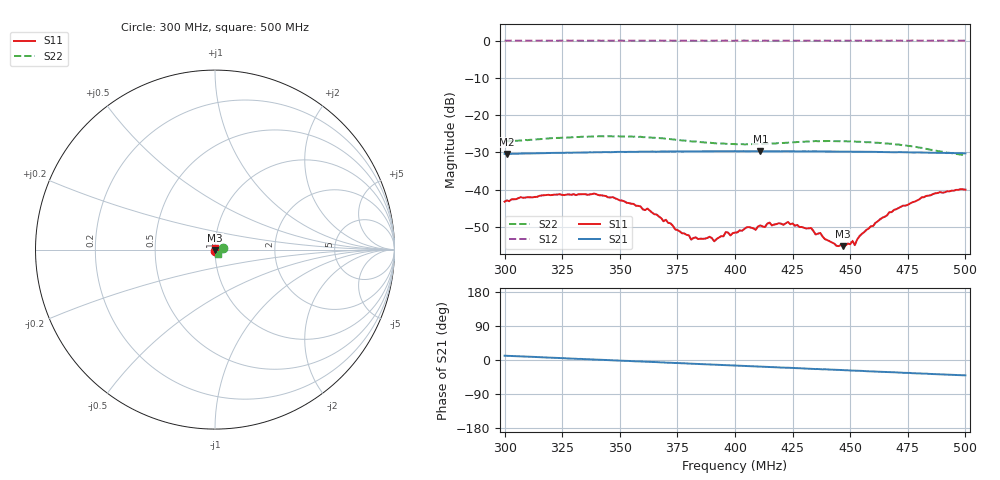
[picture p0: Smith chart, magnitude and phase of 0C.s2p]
!Prosund Technologies,SP809B,SP82221046,V.03.04.C
!Date: Monday, March 31, 2025 16:30:52
!Correction: S11(C* 2-Port  )
!S21(C* 2-Port  )
!S12(C* 2-Port  )
!S22(C* 2-Port  )
!S2P File: Measurement: :
# Hz S  dB  R 50
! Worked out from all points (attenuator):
!   201 points, 300 MHz to 500 MHz, reference 50 ohm
!   highest |S21| = -29.66 dB at 411 MHz (marker M1); lowest = -30.4 dB at 301 MHz (marker M2)
!   lowest |S11| = -55.2 dB at 447 MHz (marker M3), VSWR 1.00, Z = 50.1 - j0.142 ohm
!   |S11| at or under -10 dB: start of sweep to end of sweep
!   |S22| runs from -30.7 to -25.6 dB; largest |S21 - S12| = 0.98
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3e8  -43.21 -67.1  -30.41 11.3  0.01 0.0  -27.03 11.2
3.01e8  -42.88 -68.4  -30.41 11.1  -0.01 0.3  -27.01 10.9
3.34e8  -41.22 -52.1  -30.02 2.4  -0.02 0.1  -25.77 -0.6
3.47e8  -41.99 -32.2  -29.91 -0.9  -0.03 -0.0  -25.69 -1.5
3.62e8  -45.06 -2.5  -29.80 -4.7  -0.02 -0.2  -25.95 -2.8
3.67e8  -47.22 5.8  -29.78 -6.1  0.03 0.1  -26.15 -3.4
3.81e8  -53.41 58.6  -29.72 -9.7  -0.01 -0.3  -27.02 -8.0
3.89e8  -52.64 96.4  -29.70 -11.8  -0.00 -0.2  -27.38 -12.6
3.91e8  -53.87 111.7  -29.72 -12.2  -0.03 -0.0  -27.53 -13.7
3.96e8  -51.37 134.0  -29.66 -13.5  0.04 -0.1  -27.70 -17.0
3.98e8  -52.28 140.2  -29.69 -14.1  -0.01 -0.0  -27.74 -17.8
4e8  -51.50 151.0  -29.66 -14.7  -0.01 -0.2  -27.79 -19.4
4.11e8  -49.61 -178.0  -29.66 -17.5  0.04 0.1  -27.69 -26.9
4.23e8  -48.66 -144.9  -29.70 -20.4  0.01 0.0  -27.38 -32.4
4.34e8  -51.06 -132.5  -29.70 -23.6  -0.01 0.0  -27.00 -35.5
4.47e8  -55.17 -54.5  -29.78 -26.7  0.01 -0.0  -27.02 -36.1
4.51e8  -53.72 -28.8  -29.80 -27.9  -0.00 -0.1  -27.05 -35.9
4.52e8  -54.89 -16.2  -29.78 -28.0  0.01 0.0  -27.10 -35.9
4.55e8  -51.90 -1.7  -29.81 -28.7  0.01 -0.0  -27.19 -35.8
4.67e8  -46.05 41.9  -29.90 -32.1  -0.04 0.1  -27.64 -36.9
4.83e8  -41.68 66.7  -30.06 -35.9  0.00 -0.1  -29.04 -40.5
5e8  -40.00 87.7  -30.27 -40.6  0.03 -0.2  -30.72 -49.3
